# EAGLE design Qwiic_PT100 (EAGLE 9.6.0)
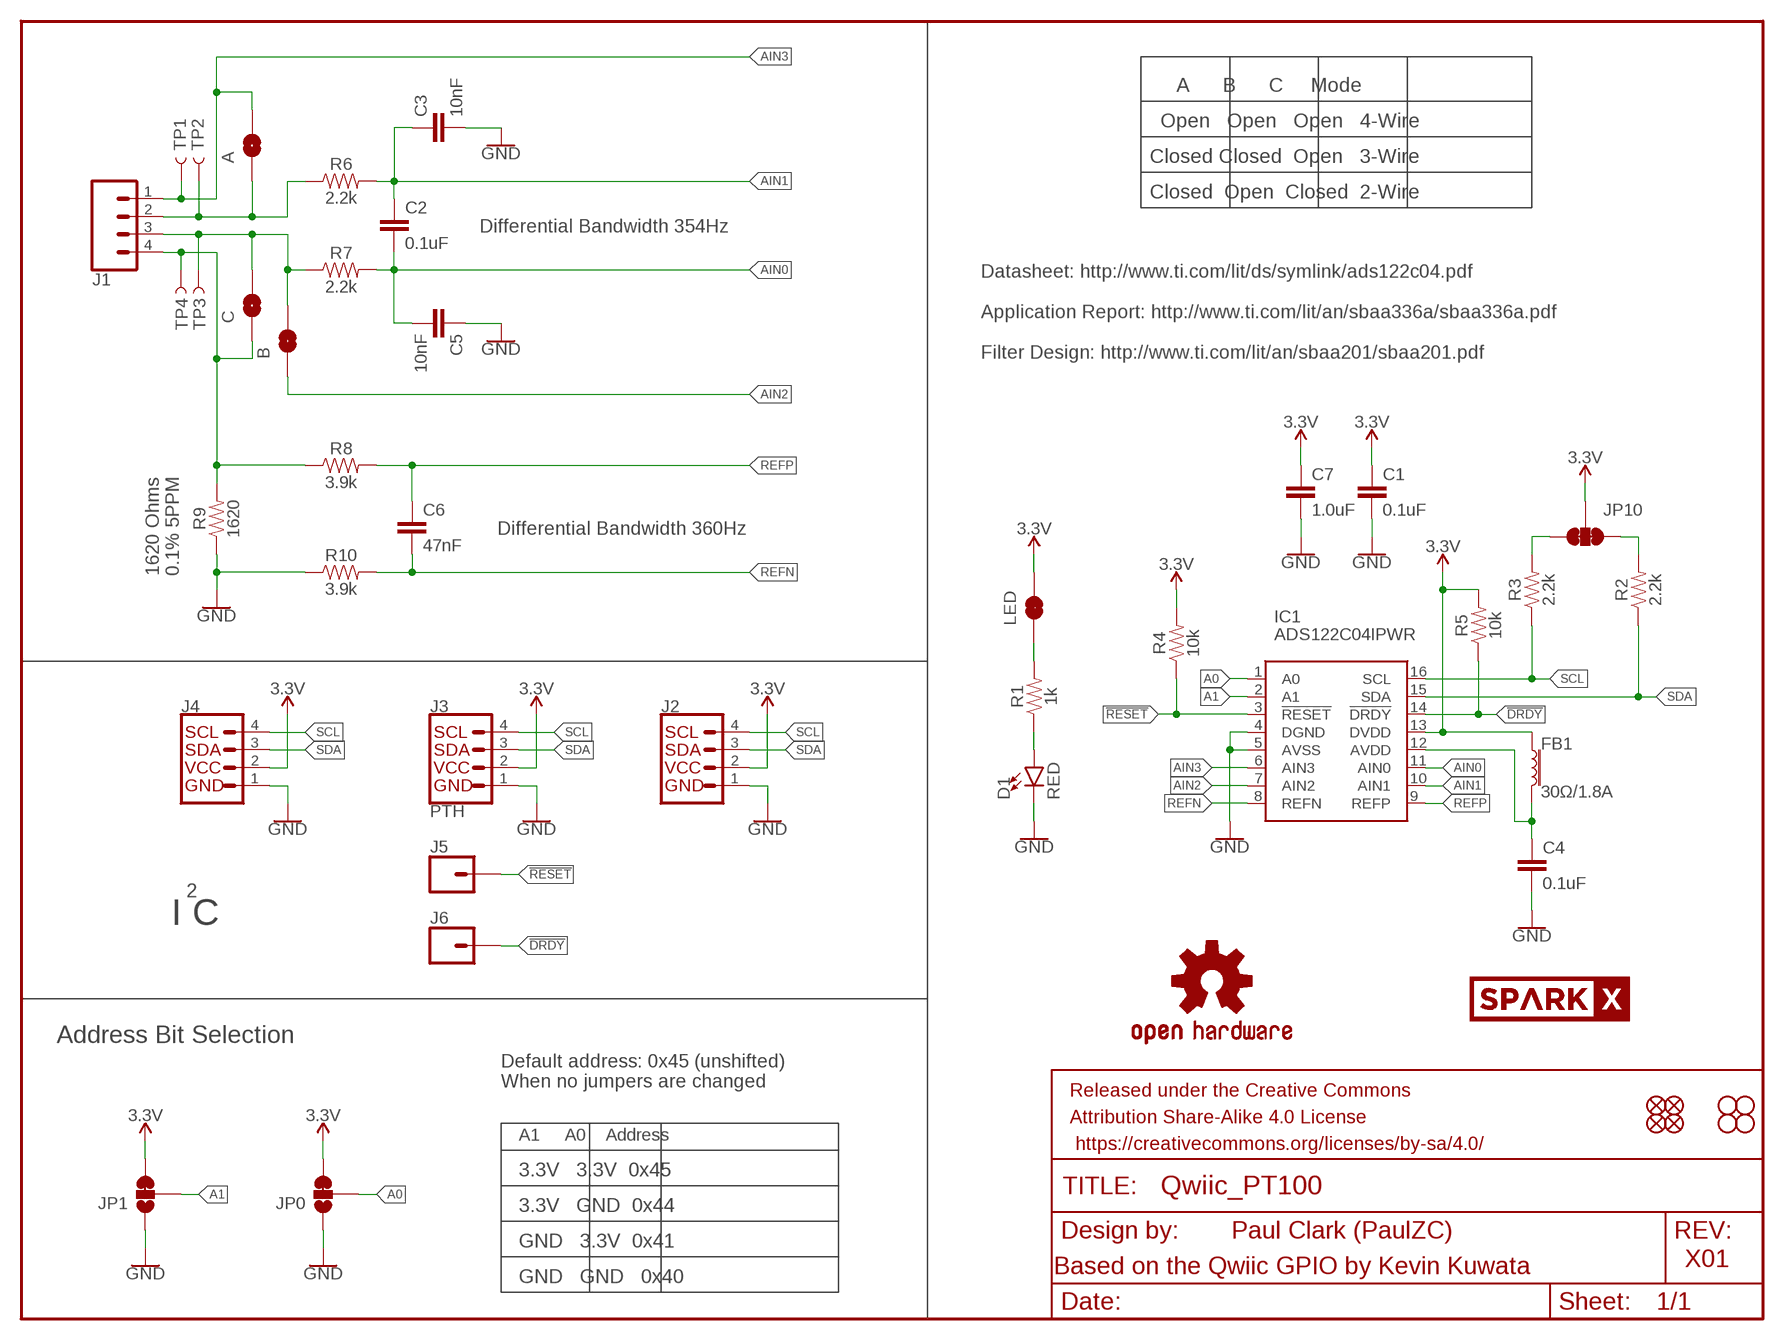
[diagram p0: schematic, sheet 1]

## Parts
A  JUMPER-SMT_2_NO_SILK_ROUND  [SMT-JUMPER_2_NO_SILK_ROUND]
B  JUMPER-SMT_2_NO_SILK_ROUND  [SMT-JUMPER_2_NO_SILK_ROUND]
C  JUMPER-SMT_2_NO_SILK_ROUND  [SMT-JUMPER_2_NO_SILK_ROUND]
C1  0.1uF  0.1UF-0603-25V-(+80/-20%)  [0603]
C2  0.1uF  0.1UF-0603-25V-5%  [0603]
C3  10nF  10NF-0603-50V-10%  [0603]
C4  0.1uF  0.1UF-0603-25V-(+80/-20%)  [0603]
C5  10nF  10NF-0603-50V-10%  [0603]
C6  47nF  47NF-0603-25V-5%  [0603]
C7  1.0uF  1.0UF-0603-16V-10%-X7R  [0603]
D1  RED  LED-RED0603  [LED-0603]
FB1  30Ω/1.8A  FERRITE_BEAD-0603  [0603]
FD1  FIDUCIAL1X2  [FIDUCIAL-1X2]
FD2  FIDUCIAL1X2  [FIDUCIAL-1X2]
FRAME1  FRAME-LETTER  [CREATIVE_COMMONS]
H1  STAND-OFF  [STAND-OFF]
H2  STAND-OFF  [STAND-OFF]
IC1  ADS122C04IPWR  [SOP65P640X120-16N]
J1  CONN_04LATCH  [LATCHTERMINAL-5MM-4]
J2  QWIIC_RIGHT_ANGLE  QWIIC_CONNECTORJS-1MM  [JST04_1MM_RA]
J3  PTH  I2C_STANDARD_NO_SILK  [1X04_NO_SILK]
J4  QWIIC_RIGHT_ANGLE  QWIIC_CONNECTORJS-1MM  [JST04_1MM_RA]
J5  CONN_01PTH_NO_SILK_YES_STOP  [1X01_NO_SILK]
J6  CONN_01PTH_NO_SILK_YES_STOP  [1X01_NO_SILK]
JP0  JUMPER-SMT_3_1-NC_TRACE_SILK  [SMT-JUMPER_3_1-NC_TRACE_SILK]
JP1  JUMPER-SMT_3_1-NC_TRACE_SILK  [SMT-JUMPER_3_1-NC_TRACE_SILK]
JP2  FIDUCIAL1X2  [FIDUCIAL-1X2]
JP3  STAND-OFF  [STAND-OFF]
JP4  STAND-OFF  [STAND-OFF]
JP6  FIDUCIAL1X2  [FIDUCIAL-1X2]
JP10  JUMPER-SMT_3_2-NC_TRACE_SILK  [SMT-JUMPER_3_2-NC_TRACE_SILK]
LED  JUMPER-SMT_2_NC_TRACE_SILK  [SMT-JUMPER_2_NC_TRACE_SILK]
LOGO1  OSHW-LOGOMINI  [OSHW-LOGO-MINI]
R1  1k  1KOHM-0603-1/10W-1%  [0603]
R2  2.2k  2.2KOHM-0603-1/10W-1%  [0603]
R3  2.2k  2.2KOHM-0603-1/10W-1%  [0603]
R4  10k  10KOHM-0603-1/10W-1%  [0603]
R5  10k  10KOHM-0603-1/10W-1%  [0603]
R6  2.2k  2.2KOHM-0603-1/10W-1%  [0603]
R7  2.2k  2.2KOHM-0603-1/10W-1%  [0603]
R8  3.9k  3.9KOHM-0603-1/10W-1%  [0603]
R9  1620  RESISTOR0603  [0603]
R10  3.9k  3.9KOHM-0603-1/10W-1%  [0603]
TP1  TEST-POINTTP_15TH_THRU  [TP_15TH]
TP2  TEST-POINTTP_15TH_THRU  [TP_15TH]
TP3  TEST-POINTTP_15TH_THRU  [TP_15TH]
TP4  TEST-POINTTP_15TH_THRU  [TP_15TH]
U$1  SPARKX-LOGO3  [SPARKX-SMALL]
U$2  SPARKX-LOGO3  [SPARKX-SMALL]

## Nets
3.3V: C1.1 C7.1 FB1.1 IC1.13(DVDD) J2.2 J3.2 J4.2 JP0.3 JP1.3 JP10.2 LED.2 R4.2 R5.2
!DRDY: IC1.14(!DRDY) J6.1 R5.1
!RESET: IC1.3(!RESET) J5.1 R4.1
A0: IC1.1(A0) JP0.2
A1: IC1.2(A1) JP1.2
AIN0: C2.2 C5.2 IC1.11(AIN0) R7.2
AIN1: C2.1 C3.1 IC1.10(AIN1) R6.2
AIN2: B.1 IC1.7(AIN2)
AIN3: A.2 IC1.6(AIN3) J1.1 TP1.P$1
GND: C1.2 C3.2 C4.2 C5.1 C7.2 D1.C IC1.4(DGND) IC1.5(AVSS) J2.1 J3.1 J4.1 JP0.1 JP1.1 R9.1 R10.1
N$1: A.1 J1.2 R6.1 TP2.P$1
N$2: D1.A R1.1
N$3: LED.1 R1.2
N$4: C4.1 FB1.2 IC1.12(AVDD)
N$5: B.2 C.2 J1.3 R7.1 TP3.P$1
N$6: C.1 J1.4 R8.1 R9.2 TP4.P$1
REFN: C6.2 IC1.8(REFN) R10.2
REFP: C6.1 IC1.9(REFP) R8.2
SCL: IC1.16(SCL) J2.4 J3.4 J4.4 R3.1
SCL_PU1: JP10.1 R2.2
SDA: IC1.15(SDA) J2.3 J3.3 J4.3 R2.1
SDA_PU1: JP10.3 R3.2

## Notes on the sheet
- A      B      C     Mode
- Open   Open   Open   4-Wire
- Closed Closed  Open   3-Wire
- Closed  Open  Closed  2-Wire
- Differential Bandwidth 354Hz
- Datasheet: http://www.ti.com/lit/ds/symlink/ads122c04.pdf
  
  Application Report: http://www.ti.com/lit/an/sbaa336a/sbaa336a.pdf
  
  Filter Design: http://www.ti.com/lit/an/sbaa201/sbaa201.pdf
- Differential Bandwidth 360Hz
- 1620 Ohms
  0.1% 5PPM
- 2
- I C
- Address Bit Selection
- Default address: 0x45 (unshifted)
  When no jumpers are changed
- A1     A0    Address
- 3.3V   3.3V  0x45
- 3.3V   GND  0x44
- Paul Clark (PaulZC)
- GND   3.3V  0x41
- X01
- Based on the Qwiic GPIO by Kevin Kuwata
- GND   GND   0x40

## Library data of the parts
A B C = SparkFun-Jumpers:JUMPER-SMT_2_NO: Normally open jumper
C1 C4 = SparkFun-Capacitors:0.1UF: 0.1µF ceramic capacitors; PROD_ID: CAP-00810
C2 = SparkFun-Capacitors:0.1UF: 0.1µF ceramic capacitors; PROD_ID: CAP-08604
C3 C5 = SparkFun-Capacitors:10NF: 0.01uF/10nF/10,000pF ceramic capacitors; PROD_ID: CAP-00867
C6 = SparkFun-Capacitors:47NF: 47nF ceramic capacitors; PROD_ID: CAP-08605
C7 = SparkFun-Capacitors:1.0UF: 1µF ceramic capacitors; PROD_ID: CAP-13930
D1 = SparkFun-LED:LED-RED: Red SMD LED; PROD_ID: DIO-00819
FB1 = SparkFun-Coils:FERRITE_BEAD: Ferrite Bead (blocks, cores, rings, chokes, etc.); PROD_ID: NDUC-13805
FD1 FD2 JP2 JP6 = SparkFun-Aesthetics:FIDUCIAL: Fiducial Alignment Points
FRAME1 = SparkFun-Aesthetics:FRAME-LETTER: Schematic Frame - Letter
H1 H2 JP3 JP4 = SparkFun-Hardware:STAND-OFF: Stand Off
IC1 = New_Parts:ADS122C04IPWR: 24-Bit, 2kSPS, 4-Ch, Low-Power Delta-Sigma ADC With PGA, Voltage Reference, IDACs and I2C Interface Source: Datasheet; HEIGHT: 1.2mm; MANUFACTURER_NAME: Texas Instruments; MANUFACTURER_PART_NUMBER: ADS122C04IPWR; MOUSER_PART_NUMBER: 595-ADS122C04IPWR
J1 = SparkFun-Connectors:CONN_04: Multi connection point. Often used as Generic Header-pin footprint for 0.1 inch spaced/style header connections On any of the 0.1 inch spaced packages, you can populate with these: Break Away Headers - Straight (PRT-00116) Break Away Male Headers - Right Angle (PRT-00553) Female Headers (PRT-00115)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; PROD_ID: CON-14722
J2 J4 = SparkFun-Connectors:QWIIC_CONNECTOR: SparkFun I2C Standard Qwiic Connector An SMD 1mm pitch JST connector makes it easy and quick (get it? Qwiic?) to connect I2C devices to each other. The Qwiic system enables fast and solderless connection between popular platforms and various sensors and actuators. We carry 200mm, 100mm, 50mm, and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; PROD_ID: CONN-13694
J3 = SparkFun-Connectors:I2C_STANDARD: SparkFun I2C Standard Pinout Header SparkFun has standardized on a pinout for all I2C based sensor breakouts. This pinout allows I2C boards to be plugged directly into the headers on Arduino Uno compatible boards, and to be daisy chained easily. Example SparkFun Products: SparkFun Atmospheric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
J5 J6 = SparkFun-Connectors:CONN_01: Single connection point. Often used as Generic Header-pin footprint for 0.1 inch spaced/style header connections
JP0 JP1 = SparkFun-Jumpers:JUMPER-SMT_3_1-NC_TRACE: Normally closed trace jumper (1 of 2 connections) This jumper has a trace between two pads so it's normally closed (NC). The other connection is normally open (NO). Use a razor knife to open the connection. For best results follow the IPC guidelines for cutting traces: Cutout at least 0.063 mm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
JP10 = SparkFun-Jumpers:JUMPER-SMT_3_2-NC_TRACE: Normally closed trace jumper (2 of 2 connections) This jumper has a trace between all three pads so they are normally closed (NC). Use a razor knife to open the connection(s). For best results follow the IPC guidelines for cutting traces: Cutout at least 0.063 mm (0.005 in). Remove all loose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
LED = SparkFun-Jumpers:JUMPER-SMT_2_NC_TRACE: Normally closed trace jumper
LOGO1 = SparkFun-Aesthetics:OSHW-LOGO: Open-Source Hardware (OSHW) Logo
R1 = SparkFun-Resistors:1KOHM: 1kΩ resistor; PROD_ID: RES-07856
R2 R3 R6 R7 = SparkFun-Resistors:2.2KOHM: 2.2kΩ resistor; PROD_ID: RES-08272
R4 R5 = SparkFun-Resistors:10KOHM: 10kΩ resistor; PROD_ID: RES-00824
R8 R10 = SparkFun-Resistors:3.9KOHM: 3.9kΩ resistor; PROD_ID: RES-08701
R9 = New_Parts:RESISTOR: Generic Resistor Package; MOUSER_PART: 660-RN731JTTD1621B05; TEMP_COEFF: 5PPM; TOLERANCE: 0.1%
TP1-TP4 = SparkFun-Connectors:TEST-POINT: SparkFun Test Points
U$1 U$2 = SparkX:SPARKX-LOGO

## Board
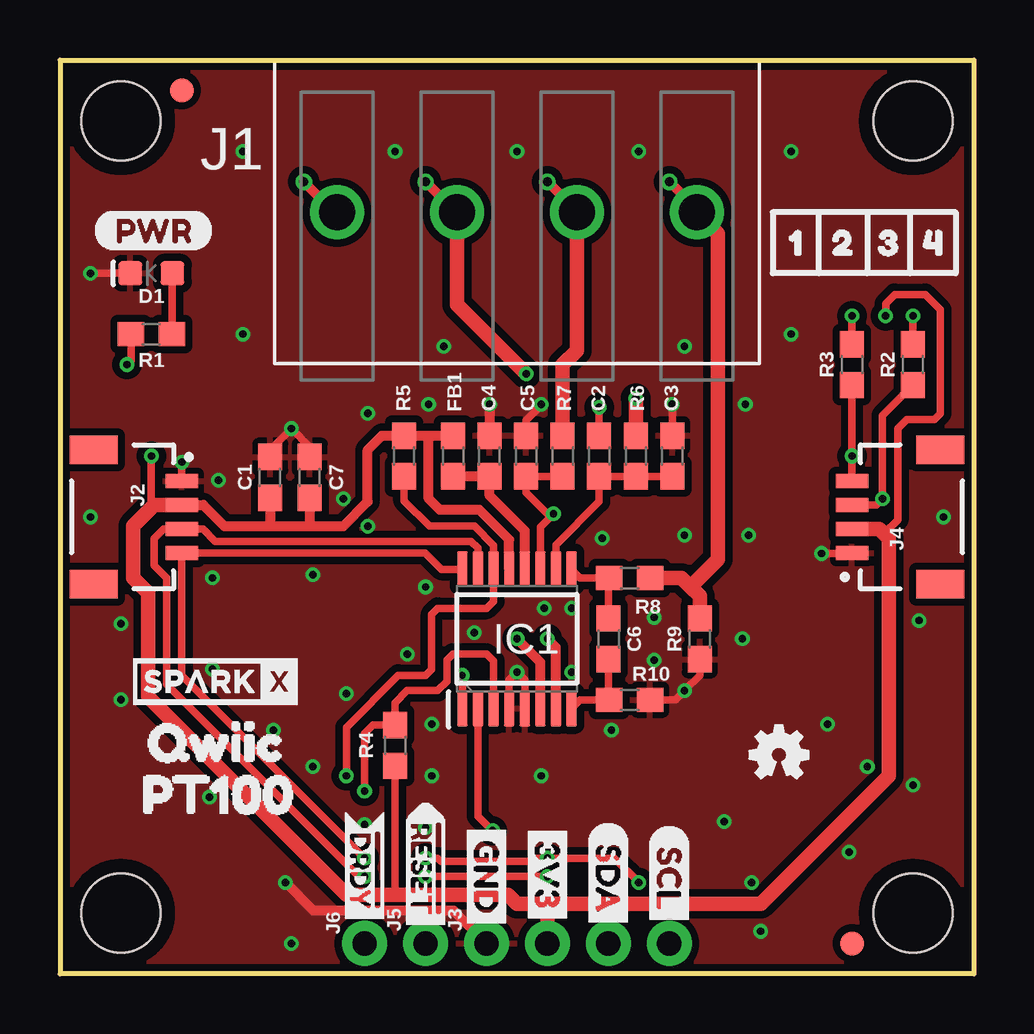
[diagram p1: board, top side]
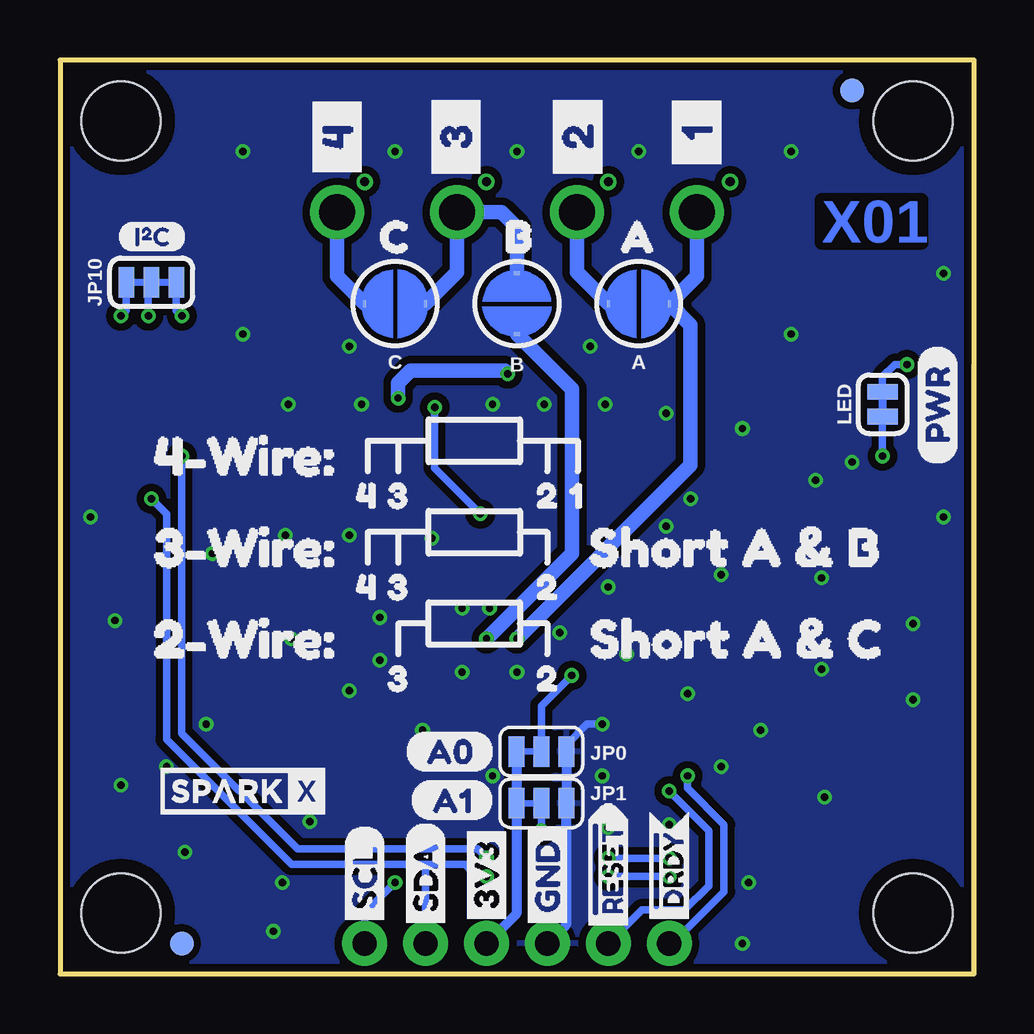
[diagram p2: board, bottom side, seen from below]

Size 38.1 x 38.1 mm. Coordinates in mm from the lower left corner, seen from the top.
Outline: 0,38.1 38.1,38.1 38.1,0 0,0 0,38.1
Copper layers (1*16): Top 0.035mm / dielectric 1.5mm / Bottom 0.035mm
Design rules "SparkFun-2-layer-PCBWay-LIMIT": minimum track width 6mil, minimum drill 0.3mm, track to track 6mil, track to pad 6mil, pad to pad 6mil, via to via 6mil, smd to smd 6mil, copper to edge 6mil, drill to drill 6mil, minimum pad ring 6mil, minimum via ring 6mil, stop-mask expansion 4mil, vias tented up to drill 25mil, thermal gap 10mil

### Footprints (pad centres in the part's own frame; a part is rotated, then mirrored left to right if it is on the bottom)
SMT-JUMPER_2_NO_SILK_ROUND = smd 0.152 x 0.305: 1 -1.27,0; 2 1.27,0
0603 = smd 1.1 x 1: 1 -0.85,0; 2 0.85,0
LED-0603 = smd 1 x 1: A -0.877,0; C 0.877,0
FIDUCIAL-1X2 = smd 1 x 1: 1 0,0
STAND-OFF = hole 3.302: 0,0
SOP65P640X120-16N = smd 1.5 x 0.45: 1 -2.9,2.275; 2 -2.9,1.625; 3 -2.9,0.975; 4 -2.9,0.325; 5 -2.9,-0.325; 6 -2.9,-0.975; 7 -2.9,-1.625; 8 -2.9,-2.275; 9 2.9,-2.275; 10 2.9,-1.625; 11 2.9,-0.975; 12 2.9,-0.325; 13 2.9,0.325; 14 2.9,0.975; 15 2.9,1.625; 16 2.9,2.275
LATCHTERMINAL-5MM-4 = drill 1.5: 1 -7.5,0; 2 -2.5,0; 3 2.5,0; 4 7.5,0
JST04_1MM_RA = smd 0.6 x 1.35: 1 -1.5,0; 2 -0.5,0; 3 0.5,0; 4 1.5,0 | smd 1.2 x 2: NC1 2.8,-3.675; NC2 -2.8,-3.675
1X04_NO_SILK = drill 1.016 pad 1.88: 1 0,0; 2 2.54,0; 3 5.08,0; 4 7.62,0
1X01_NO_SILK = drill 1.016 pad 1.88: 1 0,0
SMT-JUMPER_3_1-NC_TRACE_SILK = smd 0.66 x 1.27: 1 -1.041,0; 2 0,0; 3 1.041,0
SMT-JUMPER_3_2-NC_TRACE_SILK = smd 0.66 x 1.27: 1 -1.041,0; 2 0,0; 3 1.041,0
SMT-JUMPER_2_NC_TRACE_SILK = smd 0.66 x 1.27: 1 -0.521,0; 2 0.521,0
TP_15TH = drill 0.381 pad 0.61: P$1 0,0

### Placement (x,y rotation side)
A  13.97,27.94 0 bottom
B  19.05,27.94 90 bottom
C  24.13,27.94 0 bottom
C1  8.76,20.7 90 top
C2  22.48,21.59 90 top
C3  25.53,21.59 90 top
C4  17.91,21.59 90 top
C5  19.43,21.59 270 top
C6  22.86,13.97 270 top
C7  10.41,20.7 90 top
D1  3.81,29.21 180 top
FB1  16.38,21.59 270 top
FD1  5.08,36.83 0 bottom
FD2  33.02,1.27 270 bottom
FRAME1  not placed on the board
H1  35.56,35.56 0 top
H2  2.54,35.56 0 top
IC1  19.05,13.97 90 top
J1  19.05,31.75 0 top
J2  5.08,19.05 270 top
J3  17.78,1.27 0 top
J4  33.02,19.05 90 top
J5  15.24,1.27 0 top
J6  12.7,1.27 0 top
JP0  18.03,9.27 180 bottom
JP1  18.03,7.11 180 bottom
JP2  33.02,1.27 0 top
JP3  2.54,2.54 0 top
JP4  35.56,2.54 0 top
JP6  5.08,36.83 0 top
JP10  34.29,28.83 0 bottom
LED  3.81,23.75 270 bottom
LOGO1  29.97,9.14 0 top
R1  3.81,26.67 180 top
R2  35.56,25.4 90 top
R3  33.02,25.4 90 top
R4  13.97,9.53 270 top
R5  14.35,21.59 90 top
R6  24,21.59 270 top
R7  20.95,21.59 270 top
R8  23.75,16.51 180 top
R9  26.67,13.97 90 top
R10  23.75,11.43 180 top
TP1  10.16,33.02 0 top
TP2  15.24,33.02 0 top
TP3  20.32,33.02 0 top
TP4  25.4,33.02 0 top
U$1  30.48,7.62 0 bottom
U$2  6.48,12.19 0 top
U$3  [3V33]  20.32,6.48 270 top
U$4  [_1_0]  11.56,33.15 90 bottom
U$5  [A11]  23.5,7.24 0 bottom
U$6  [_2_0]  16.51,32.77 90 bottom
U$7  [GND4]  17.78,6.48 270 top
U$8  [PT1000]  2.03,7.49 0 top
U$9  [SCL6]  25.4,6.22 270 top
U$10  [SDA5]  22.86,6.35 270 top
U$11  [A00]  23.75,9.27 0 bottom
U$12  [_3_0]  21.59,32.77 90 bottom
U$13  [_4_0]  26.54,32.77 90 bottom
U$14  [#DRDY0]  12.7,6.99 270 top
U$15  [#DRDY0]  12.7,1.65 90 bottom
U$16  [#RESET0]  15.24,7.37 270 top
U$17  [#RESET0]  15.24,1.4 90 bottom
U$18  [A0]  15.88,30.73 0 bottom
U$19  [B0]  20.7,30.73 0 bottom
U$20  [I_SUPER2_C-()-03]  35.69,30.73 0 bottom
U$21  [40]  35.05,30.48 0 top
U$22  [C0]  25.91,30.73 0 bottom
U$23  [SCL0]  25.4,1.78 90 bottom
U$24  [SDA1]  22.86,1.65 90 bottom
U$25  [GND4]  17.78,1.65 90 bottom
U$26  [3V33]  20.32,1.78 90 bottom
U$27  [31]  33.02,30.48 0 top
U$28  [20]  31.11,30.48 0 top
U$29  [15]  17.78,19.94 0 bottom
U$30  [40]  26.67,19.94 0 bottom
U$31  [2#WIRE#0]  35.56,13.97 0 bottom
U$32  [QWIIC1]  2.29,9.65 0 top
U$33  [20]  19.3,19.94 0 bottom
U$34  [31]  25.53,19.94 0 bottom
U$35  [15]  29.46,30.48 0 top
U$36  [3#WIRE#0]  35.56,17.78 0 bottom
U$37  [20]  19.3,16.13 0 bottom
U$38  [31]  25.53,16.13 0 bottom
U$39  [PWR0]  1.4,30.99 0 top
U$40  [PWR0]  1.52,21.21 90 bottom
U$41  [4#WIRE#0]  35.56,21.59 0 bottom
U$42  [SHORT_A_#_B0]  17.4,17.78 0 bottom
U$43  [SHORT_A_#_C0]  17.4,13.97 0 bottom
U$44  [40]  26.67,16.13 0 bottom
U$46  [20]  19.3,12.32 0 bottom
U$47  [31]  25.53,12.32 0 bottom

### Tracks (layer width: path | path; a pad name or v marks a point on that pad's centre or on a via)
3.3V  (via drill 0.3)
  Top 0.305: v34.42,27.43 34.42,27.94 34.8,28.32 36.07,28.32 36.7,27.69 36.7,23.37 36.45,23.11 35.31,23.11 34.92,22.73 34.92,18.92 34.35,18.35 | R4.2 13.97,3.3 | v3.81,21.59 3.81,19.67 3.93,19.55
  Top 0.406: 10.41,18.66 11.8,18.66 12.83,19.68 12.83,21.84 13.42,22.44 R5.2 15.37,22.44 | 10.41,18.66 8.76,18.66 | 8.76,18.66 6.86,18.66 5.97,19.55 J2.2 | C1.1 8.76,18.66 | C7.1 10.41,18.66 | IC1.13 18.73,18.11 17.49,19.34 15.84,19.34 15.37,19.81 15.37,22.44 | 15.37,22.44 FB1.1
  Top 0.61: J3.2 20.32,2.92 | J2.2 3.93,19.55 3.05,18.67 3.05,16.51 3.68,15.88 3.68,11.56 11.94,3.3 13.97,3.3 18.67,3.3 19.05,2.92 20.32,2.92 | J4.2 34.16,18.55 34.35,18.35 34.54,18.16 34.54,8.26 29.21,2.92 20.32,2.92
  Bottom 0.305: LED.2 v3.81,21.59 | JP10.2 34.42,28.7 v34.42,27.43
  Bottom 0.406: J3.2 19.07,2.52 JP1.3 JP0.3
!DRDY  (via drill 0.3)
  Top 0.305: R5.1 14.35,19.72 15.41,18.67 17.27,18.67 18.07,17.87 IC1.14 18.07,15.54 17.78,15.24 15.75,15.24 15.49,14.99 15.49,12.7 15.24,12.45 14.1,12.45 11.94,10.29 v11.94,8.26
  Bottom 0.305: J6.1 12.57,1.27 10.41,3.43 10.41,6.22 11.94,7.75 v11.94,8.26
!RESET  (via drill 0.3)
  Top 0.305: IC1.3 18.07,13.04 17.78,13.34 16.38,13.34 16.13,13.08 16.13,12.19 15.75,11.81 14.48,11.81 13.97,11.3 R4.1 13.04,10.38 12.7,10.03 v12.7,7.62
  Bottom 0.305: v12.7,7.62 11.05,5.97 11.05,3.68 12.06,2.67 13.84,2.67 J5.1
A0  (via drill 0.3)
  Top 0.305: 16.77,12.44 IC1.1
  Top 0.406: v16.76,12.45 16.77,12.44
  Bottom 0.305: JP0.2 18.03,11.18 v16.76,12.45
A1  (via drill 0.3)
  Top 0.305: v18.03,5.97 17.43,6.58 IC1.2
  Bottom 0.305: JP1.2 v18.03,5.97
AIN0  (via drill 0.3)
  Top 0.305: R7.2 C5.2 19.43,20.07 20.32,19.18 v20.57,19.18 20.02,18.63 IC1.11 | v22.48,23.62 C2.2
  Bottom 0.305: v20.57,19.18 22.48,21.08 v22.48,23.62
AIN1
  Top 0.305: IC1.10 20.68,17.88 22.48,19.68 C2.1 R6.2 C3.1
AIN2  (via drill 0.3)
  Top 0.406: IC1.7 20.68,13.62 v20.32,13.97
  Bottom 0.61: B.1 16.76,24.38 16.76,17.53 v20.32,13.97
AIN3  (via drill 0.3)
  Top 0.406: IC1.6 20.02,12.99 v19.05,13.97 | TP1.P$1 11.43,31.75 J1.1
  Bottom 0.61: J1.1 11.55,29.09 A.2 11.81,27.05 11.81,21.21 v19.05,13.97
GND  (via drill 0.3)
  Top 0.305: IC1.4 18.73,12.25 v19.05,12.57 19.38,12.25 IC1.5 | C7.2 10.41,21.97 v9.65,22.73 8.76,21.84 C1.2 | v1.27,29.21 D1.C | J2.1 v5.08,21.34 | J4.1 33,17.53 v31.75,17.53 | v20.07,23.75 20.07,23.71 19.43,23.07 C5.1 | C3.2 v25.53,23.75 | R10.1 25.65,11.43 v26.04,11.81 26.67,12.45 R9.1
  Top 0.406: v17.91,23.75 C4.2 | J3.1 16.41,2.64 10.57,2.64 v9.4,3.81
  Bottom 0.305: JP0.1 16.99,9.55 16.13,10.41 v15.49,10.41
  Bottom 0.406: J3.1 16.99,2.06 JP1.1 JP0.1
  other vias: 28.83,3.81 33.66,8.64 27.69,6.35 32,10.41 29.21,1.78 32.89,5.08 35.56,7.87 2.54,11.43 6.22,7.37 8.89,10.16 6.35,12.7 10.54,8.64 6.35,16.51 15.24,16.13 20.19,15.24 21.34,15.24 21.34,12.57 24.77,14.86 24.77,13.08 2.54,14.61 1.27,19.05 6.6,20.57 11.81,19.81 12.83,18.67 12.83,23.37 36.83,19.05 17.27,14.22 14.48,13.34 10.54,16.64 11.94,11.68 22.61,18.16 26.04,18.29 28.7,18.29 28.57,23.75 15.37,23.75 13.97,34.29 19.05,34.29 24.13,34.29 30.48,34.29 30.48,26.67 7.62,26.67 7.62,34.29 16,26.16 26.04,26.16 15.24,6.1 12.7,6.22 20.07,8.26 22.99,10.16 28.45,13.97 35.81,14.73 15.49,8.26 9.65,1.27
  pour Top (isolate 0.305): 0,38.1 38.1,38.1 38.1,0 0,0
  pour Bottom (isolate 0.305): 0,38.1 38.1,38.1 38.1,0 0,0
N$1  (via drill 0.3)
  Top 0.406: TP2.P$1 16.51,31.75 J1.2
  Top 0.61: J1.2 16.55,27.9 v19.43,25.02 | v24,24 R6.1
  Bottom 0.61: A.1 16.55,29.25 J1.2 | v19.43,25.02 19.56,25.15 23.5,25.15 24,24.64 v24,24
N$2
  Top 0.305: D1.A 4.69,26.7 R1.1
N$3  (via drill 0.3)
  Top 0.305: R1.2 2.96,25.57 v2.79,25.4
  Bottom 0.305: v2.79,25.4 3.3,25.4 3.81,24.89 LED.1
N$4
  Top 0.406: IC1.12 19.38,18.47 17.91,19.94 C4.1 FB1.2
N$5
  Top 0.406: TP3.P$1 21.55,31.79 J1.3
  Top 0.61: R7.1 20.95,25.4 21.55,26 J1.3
  Bottom 0.61: B.2 19.05,31.11 19.68,31.75 J1.3 21.55,29.25 C.2
N$6
  Top 0.406: TP4.P$1 26.55,31.87 J1.4
  Top 0.61: R8.1 25.91,16.51 26.29,16.13 | R9.2 26.67,15.75 26.29,16.13 | J1.4 27.43,30.87 27.43,17.27 26.29,16.13
  Bottom 0.61: C.1 26.55,29.09 J1.4
REFN
  Top 0.305: IC1.8 21.68,11.43 R10.2 22.86,11.47 C6.2
REFP
  Top 0.305: IC1.9 21.68,16.51 R8.2 22.86,16.47 C6.1
SCL  (via drill 0.3)
  Top 0.305: R3.1 v33.02,21.59 J4.4 | IC1.16 15.9,16.87 15.22,17.55 J2.4 5.08,12.45 v12.7,4.83 | v15.24,4.83 15.75,4.83 15.88,4.7 19.68,4.7 19.81,4.83 v20.32,4.83 23.11,4.83 v24.13,3.81
  Bottom 0.305: v12.7,4.83 v15.24,4.83 | v20.32,4.83 20.7,5.21 28.19,5.21 33.02,10.03 v33.02,21.59 | v24.13,3.81 25.4,2.54 J3.4
SCL_PU1  (via drill 0.3)
  Top 0.305: R2.2 v35.56,27.43
  Bottom 0.305: JP10.1 35.33,27.66 v35.56,27.43
SDA  (via drill 0.3)
  Top 0.305: R2.1 34.29,23.28 v34.29,19.81 34.03,19.55 J4.3 | IC1.15 17.43,17.75 17.14,18.03 6.48,18.03 5.96,18.55 J2.3 4.33,18.55 3.94,18.16 3.94,17.02 4.45,16.51 4.45,12.06 12.45,4.06 v12.7,4.06 | v20.32,4.06 v15.24,4.06
  Bottom 0.305: v15.24,4.06 v12.7,4.06 | v20.32,4.06 20.7,4.06 21.21,4.57 22.86,4.57 | 22.86,4.57 28.45,4.57 33.66,9.78 33.66,19.18 v34.29,19.81 | J3.3 22.86,4.57
SDA_PU1  (via drill 0.3)
  Top 0.305: R3.2 v33.02,27.43
  Bottom 0.305: JP10.3 33.25,27.66 v33.02,27.43

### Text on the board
Bottom: X01

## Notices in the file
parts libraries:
SparkFun-Resistors: Licensing: Creative Commons ShareAlike 4.0 International - https://creativecommons.org/licenses/by-sa/4.0
SparkFun-Aesthetics: Released under the Creative Commons Attribution Share-Alike 4.0 License
SparkFun-Aesthetics: https://creativecommons.org/licenses/by-sa/4.0
